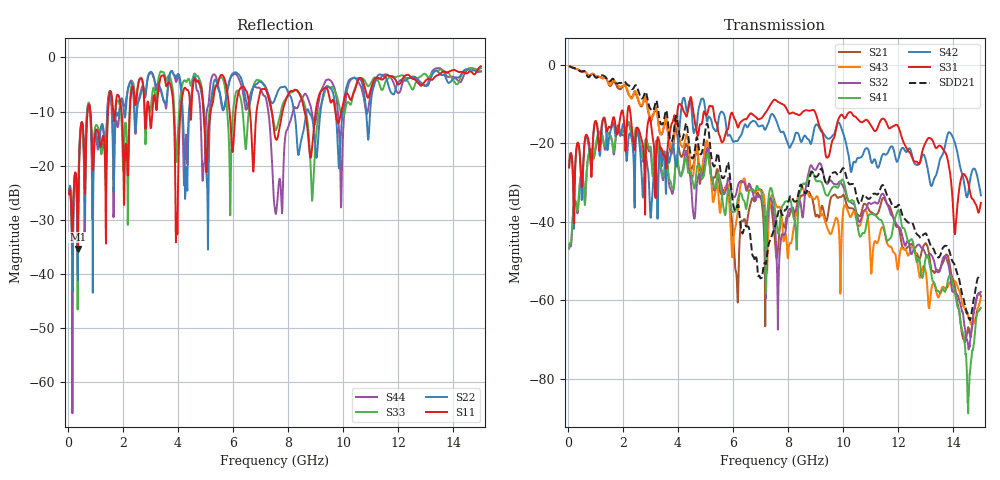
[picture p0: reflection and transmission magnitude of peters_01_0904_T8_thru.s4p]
# MHZ S RI R 50.00
! FREQ  S11  S12  S13  S14
!  S21  S22  S23  S24
!  S31  S32  S33  S34
!  S41  S42  S43  S44
!  REAL  IMAG  REAL  IMAG  REAL  IMAG  REAL  IMAG
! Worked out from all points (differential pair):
!   1496 points, 50 MHz to 15 GHz, reference 50 ohm
!   strongest paths, dB at 50 MHz, 3.79 GHz, 7.53 GHz, 11.27 GHz, 15 GHz:
!     S31: -26.2, -14.8, -8.9, -15.7, -35.2
!     S42: -26.2, -20.8, -13.6, -26.2, -33.3
!     S41: -46.7, -31.4, -37.2, -39.1, -61.9
!     S32: -46.9, -32.9, -41.1, -35.3, -57.9
!     S43: -0.4, -20.6, -35.1, -45.0, -59.5
!     S21: -0.4, -22.3, -45.6, -37.7, -59.0
!   taken as a pair (ports 3,1 in; 4,2 out), SDD21 dB: -0.3, -19.3, -41.2, -32.9, -53.5
!   lowest |S11| = -35.4 dB at 360 MHz (marker M1), VSWR 1.03, Z = 51.5 - j0.863 ohm
!   |S11| at or under -10 dB: start of sweep to 719.7 MHz; 822.1 MHz to 1.458 GHz (636.4 MHz wide, 55.8 % of centre); 8.599 GHz to 9.003 GHz (404.7 MHz wide, 4.6 % of centre)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
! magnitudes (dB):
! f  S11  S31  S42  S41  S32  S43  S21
! 50 MHz  -25.3  -26.2  -26.2  -46.7  -46.9  -0.4  -0.4
! 360 MHz  -35.4  -19.9  -20.0  -37.4  -37.8  -1.2  -1.2
! 5.05 GHz  -20.4  -12.8  -14.3  -23.0  -21.6  -19.3  -19.9
! 6.14 GHz  -8.0  -15.3  -19.4  -35.6  -32.1  -39.1  -55.0
! 7.55 GHz  -15.1  -9.0  -13.9  -38.4  -43.6  -35.5  -47.4
! 9.15 GHz  -6.6  -15.9  -16.4  -29.7  -25.1  -37.0  -38.5
! 15 GHz  -1.6  -35.2  -33.3  -61.9  -57.9  -59.5  -59.0
